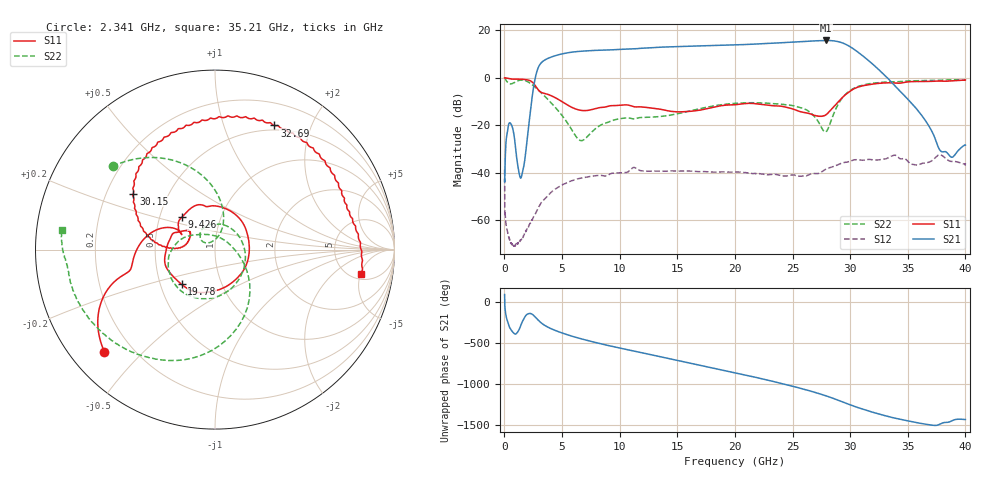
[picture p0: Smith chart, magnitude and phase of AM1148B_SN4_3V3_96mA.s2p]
!Agilent Technologies,E8363B,US42420178,A.07.50.48
!Agilent E8363B: A.07.50.48
!Date: Thursday, November 17, 2022 10:10:19
!Correction: S11(Full 2 Port(1,2))
!S21(Full 2 Port(1,2))
!S12(Full 2 Port(1,2))
!S22(Full 2 Port(1,2))
!S2P File: Measurements: S11, S21, S12, S22:
# Hz S  dB  R 50
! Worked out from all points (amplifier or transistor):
!   6401 points, 10 MHz to 40 GHz, reference 50 ohm
!   highest |S21| = 15.8 dB at 27.88 GHz (marker M1)
!   |S21| within 3 dB of that: 12.93 GHz to 30.11 GHz (17.18 GHz wide, 79.8 % of centre)
!   unconditionally stable (mu >= 1): 65.58 MHz to end of sweep
!   at 6.671 GHz: K = 17.18, MAG = 11.4 dB, |S12| = -42.4 dB
!   at 20 GHz: K = 8.43, MAG = 14.6 dB, |S12| = -39.8 dB
!   at 40 GHz: K = 32.96, MAG = -14.4 dB, |S12| = -36.0 dB
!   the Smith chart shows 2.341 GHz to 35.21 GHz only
!   S11 on the Smith chart (normalised r, x): 2.341 GHz: 0.10, -0.39; 9.426 GHz: 0.65, +0.25; 19.78 GHz: 0.64, -0.27; 30.15 GHz: 0.31, +0.28; 32.69 GHz: 0.45, +1.49; 35.21 GHz: 6.00, -5.19
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1e7  -0.01 -0.4  -43.17 93.8  -38.77 -13.7  -0.01 -2.7
2.340667e9  -1.53 -137.3  -10.39 -141.6  -60.70 -123.0  -2.67 140.9
3.665336e9  -6.84 -174.4  7.96 63.8  -50.28 152.3  -8.62 94.3
4.996253e9  -10.06 157.4  10.11 -14.7  -45.24 88.5  -15.91 73.0
6.677083e9  -13.77 155.1  11.25 -86.7  -42.34 25.6  -26.53 114.9
9.426395e9  -11.75 135.5  11.85 179.5  -40.27 -52.3  -17.90 129.3
1.334417e10  -13.13 51.7  12.89 61.5  -39.37 -164.4  -16.39 33.5
1.610598e10  -14.14 -36.9  13.38 -21.7  -39.34 117.6  -13.95 -41.2
1.803049e10  -12.61 -94.4  13.59 -79.5  -39.79 64.5  -12.00 -79.7
1.978006e10  -11.43 -133.8  13.86 -132.6  -39.82 16.4  -10.86 -108.5
2.0005e10  -11.35 -138.9  13.90 -139.4  -39.78 10.6  -10.77 -111.7
2.193577e10  -11.01 -172.4  14.31 160.1  -40.48 -41.4  -10.58 -136.7
2.393527e10  -11.95 160.0  14.80 93.6  -41.20 -99.8  -11.08 -158.8
2.520995e10  -13.51 151.1  15.12 48.6  -41.18 -140.6  -11.93 -174.9
2.667208e10  -15.43 145.3  15.56 -7.5  -40.48 163.5  -15.13 155.6
2.788428e10  -15.68 170.1  15.78 -60.1  -38.62 105.4  -22.82 55.2
2.884029e10  -10.77 176.4  15.41 -108.0  -36.90 53.9  -12.24 -39.8
3.015246e10  -5.17 145.5  12.65 -178.3  -34.93 -12.0  -4.85 -93.6
3.268933e10  -2.31 64.4  2.50 69.9  -34.48 -105.9  -1.89 -153.2
3.333917e10  -2.12 45.4  -0.56 45.7  -33.64 -123.7  -1.71 -163.4
3.520745e10  -1.65 -9.5  -10.09 -11.4  -36.18 165.1  -1.29 172.6
4e10  -0.95 -123.1  -28.38 10.4  -36.00 42.7  -1.00 118.2
